| IBIS file stm32u375_385_lqfp100.ibs
[IBIS ver] 4.2
[File name] stm32u375_385_lqfp100.ibs
[File Rev] 1.2
[Date] 23-06-2025
[Source] Data Created at STMicroelectronics
[Notes]  File originated from ELDO simulations.
[Disclaimer]  This information is for modeling purpose only and is
   not guaranted. The information is subject to change without
   notice.
[Copyright] Copyright 2025 STMicroelectronics Inc.
|   Component stm32u375_385_lqfp100
[Component] stm32u375_385_lqfp100
[Manufacturer] STMicroelectronics
[Package]
| variable   typ   min   max
R_pkg  0  NA  NA
L_pkg  0  NA  NA
C_pkg  0  NA  NA
[Pin]   signal_name   model_name
1  PE2  io8_ft_100m
2  PE3  io8_ft_100m_hslv
3  PE4  io8_ft_100m
4  PE5  io8_ft_100m
5  PE6  io8_ft_100m
6  VBAT  power
7  PC13  io8_ft_100m_v33
8  PC14-OSC32_IN  io_ft_tamp
9  PC15-OSC32_OUT  io_ft_tamp
10  VSS  gnd
11  VDD  power
12  PH0-OSC_IN  io8_ft_100m
13  PH1-OSC_OUT  io8_ft_100m
14  NRST  ioreset_v33
15  PC0  io8_ft_100m_hslv
16  PC1  io8_ft_100m_hslv
17  PC2  io8_ft_100m_hslv
18  PC3  io8_ft_100m_hslv
19  VSSA  nc
20  VREFM  nc
21  VREFP  nc
22  VDDA  nc
23  PA0  io8_ft_100m
24  PA1  io8_ft_100m_hslv
25  PA2  io8_ft_100m_hslv
26  PA3  io8_ft_100m_hslv
27  VSS  gnd
28  VDD  power
29  PA4  io8_ft_100m_hslv
30  PA5  io8_ft_100m
31  PA6  io8_ft_100m_hslv
32  PA7  io8_ft_100m_hslv
33  PC4  io8_ft_100m_hslv
34  PC5  io8_ft_100m
35  PB0  io8_ft_100m_hslv
36  PB1  io8_ft_100m_hslv
37  PB2  io8_ft_100m_hslv
38  PE7  io8_ft_100m
39  PE8  io8_ft_100m
40  PE9  io8_ft_100m_hslv
41  PE10  io8_ft_100m_hslv
42  PE11  io8_ft_100m_hslv
43  PE12  io8_ft_100m_hslv
44  PE13  io8_ft_100m_hslv
45  PE14  io8_ft_100m_hslv
46  PE15  io8_ft_100m_hslv
47  PB10  io8_ft_100m_hslv
48  VCAP  nc
49  VSS  gnd
50  VDD  power
51  PB12  io8_ft_100m_hslv
52  PB13  io8_ft_100m_hslv
53  PB14  io8_ft_100m_hslv
54  PB15  io8_ft_100m
55  PD8  io8_ft_100m
56  PD9  io8_ft_100m
57  PD10  io8_ft_100m
58  PD11  io8_ft_100m
59  PD12  io8_ft_100m_hslv
60  PD13  io8_ft_100m_hslv
61  PD14  io8_ft_100m
62  PD15  io8_ft_100m
63  PC6  io8_ft_100m_hslv
64  PC7  io8_ft_100m_hslv
65  PC8  io8_ft_100m_hslv
66  PC9  io8_ft_100m_hslv
67  PA8  io8_ft_100m_hslv
68  PA9  io8_ft_100m
69  PA10  io8_ft_100m
70  PA11  io8usb_ft_phy
71  PA12  io8usb_ft_phy
72  PA13  io8_ft_100m
73  VDDUSB  power
74  VSS  gnd
75  VDD  power
76  PA14  io8_ft_100m
77  PA15  io8_ft_100m
78  PC10  io8_ft_100m_hslv
79  PC11  io8_ft_100m_hslv
80  PC12  io8_ft_100m_hslv
81  PD0  io8_ft_100m
82  PD1  io8_ft_100m
83  PD2  io8_ft_100m_hslv
84  PD3  io8_ft_100m_hslv
85  PD4  io8_ft_100m_hslv
86  PD5  io8_ft_100m_hslv
87  PD6  io8_ft_100m_hslv
88  PD7  io8_ft_100m_hslv
89  PB3  io8_ft_100m_hslv
90  PB4  io8_ft_100m_hslv
91  PB5  io8_ft_100m_hslv
92  PB6  io8_ft_100m_hslv
93  PB7  io8_ft_100m_hslv
94  PH3-BOOT0  io8_ft_100m_hslv
95  PB8  io8_ft_100m_hslv
96  PB9  io8_ft_100m_hslv
97  PE0  io8_ft_100m
98  PE1  io8_ft_100m
99  VSS  gnd
100  VDD  power
[Package Model]   454-lqfp-14x14-100-ldo-250417
[Pin Mapping]   pulldown_ref   pullup_ref   | Comment
1  gndio  vddio
2  gndio  vddio
3  gndio  vddio
4  gndio  vddio
5  gndio  vddio
6  nc  vsw
7  gndio  vsw
8  gndio  vsw
9  gndio  vsw
10  gndio  nc
11  nc  vddio
12  gndio  vddio
13  gndio  vddio
14  gndio  vddio
15  gndio  vddio
16  gndio  vddio
17  gndio  vddio
18  gndio  vddio
19  nc  nc
20  nc  nc
21  nc  nc
22  nc  nc
23  gndio  vddio
24  gndio  vddio
25  gndio  vddio
26  gndio  vddio
27  gndio  nc
28  nc  vddio
29  gndio  vddio
30  gndio  vddio
31  gndio  vddio
32  gndio  vddio
33  gndio  vddio
34  gndio  vddio
35  gndio  vddio
36  gndio  vddio
37  gndio  vddio
38  gndio  vddio
39  gndio  vddio
40  gndio  vddio
41  gndio  vddio
42  gndio  vddio
43  gndio  vddio
44  gndio  vddio
45  gndio  vddio
46  gndio  vddio
47  gndio  vddio
48  nc  nc
49  gndio  nc
50  nc  vddio
51  gndio  vddio
52  gndio  vddio
53  gndio  vddio
54  gndio  vddio
55  gndio  vddio
56  gndio  vddio
57  gndio  vddio
58  gndio  vddio
59  gndio  vddio
60  gndio  vddio
61  gndio  vddio
62  gndio  vddio
63  gndio  vddio
64  gndio  vddio
65  gndio  vddio
66  gndio  vddio
67  gndio  vddio
68  gndio  vddio
69  gndio  vddio
70  gndio  vddusb  | Depending on IO usage
| 70  gndio  vddio  | Depending on IO usage
71  gndio  vddusb  | Depending on IO usage
| 71  gndio  vddio  | Depending on IO usage
72  gndio  vddio
73  nc  vddusb
74  gndio  nc
75  nc  vddio
76  gndio  vddio
77  gndio  vddio
78  gndio  vddio
79  gndio  vddio
80  gndio  vddio
81  gndio  vddio
82  gndio  vddio
83  gndio  vddio
84  gndio  vddio
85  gndio  vddio
86  gndio  vddio
87  gndio  vddio
88  gndio  vddio
89  gndio  vddio
90  gndio  vddio
91  gndio  vddio
92  gndio  vddio
93  gndio  vddio
94  gndio  vddio
95  gndio  vddio
96  gndio  vddio
97  gndio  vddio
98  gndio  vddio
99  gndio  nc
100  nc  vddio
|[Diff Pin]  inv_pin  vdiff  tdelay_typ  tdelay_min  tdelay_max
|71  70  NA  NA  NA  NA
[Model Selector] io8_ft_100m
io8_ft_100m_ls_1v2  "GPIO 100MHz - 5V tolerant - low speed - 1.2V range"
io8_ft_100m_ls_1v8  "GPIO 100MHz - 5V tolerant - low speed - 1.8V range"
io8_ft_100m_ls_3v3  "GPIO 100MHz - 5V tolerant - low speed - 3.3V range"
io8_ft_100m_ms_1v2  "GPIO 100MHz - 5V tolerant - med speed - 1.2V range"
io8_ft_100m_ms_1v8  "GPIO 100MHz - 5V tolerant - med speed - 1.8V range"
io8_ft_100m_ms_3v3  "GPIO 100MHz - 5V tolerant - med speed - 3.3V range"
io8_ft_100m_fs_1v2  "GPIO 100MHz - 5V tolerant - fast speed - 1.2V range"
io8_ft_100m_fs_1v8  "GPIO 100MHz - 5V tolerant - fast speed - 1.8V range"
io8_ft_100m_fs_3v3  "GPIO 100MHz - 5V tolerant - fast speed - 3.3V range"
io8_ft_100m_hs_1v2  "GPIO 100MHz - 5V tolerant - high speed - 1.2V range"
io8_ft_100m_hs_1v8  "GPIO 100MHz - 5V tolerant - high speed - 1.8V range"
io8_ft_100m_hs_3v3  "GPIO 100MHz - 5V tolerant - high speed - 3.3V range"
[Model Selector] io8_ft_100m_hslv
io8_ft_100m_ls_1v2  "GPIO 100MHz - 5V tolerant - low speed - 1.2V range"
io8_ft_100m_ls_1v8  "GPIO 100MHz - 5V tolerant - low speed - 1.8V range"
io8_ft_100m_ls_3v3  "GPIO 100MHz - 5V tolerant - low speed - 3.3V range"
io8_ft_100m_ms_1v2  "GPIO 100MHz - 5V tolerant - med speed - 1.2V range"
io8_ft_100m_ms_1v8  "GPIO 100MHz - 5V tolerant - med speed - 1.8V range"
io8_ft_100m_ms_3v3  "GPIO 100MHz - 5V tolerant - med speed - 3.3V range"
io8_ft_100m_fs_1v2  "GPIO 100MHz - 5V tolerant - fast speed - 1.2V range"
io8_ft_100m_fs_1v8  "GPIO 100MHz - 5V tolerant - fast speed - 1.8V range"
io8_ft_100m_fs_3v3  "GPIO 100MHz - 5V tolerant - fast speed - 3.3V range"
io8_ft_100m_hs_1v2  "GPIO 100MHz - 5V tolerant - high speed - 1.2V range"
io8_ft_100m_hs_1v8  "GPIO 100MHz - 5V tolerant - high speed - 1.8V range"
io8_ft_100m_hs_3v3  "GPIO 100MHz - 5V tolerant - high speed - 3.3V range"
io8_ft_100m_hslv_ls_1v2  "GPIO 100MHz low voltage optimization - 5V tolerant - low speed - 1.2V range"
io8_ft_100m_hslv_ls_1v8  "GPIO 100MHz low voltage optimization - 5V tolerant - low speed - 1.8V range"
io8_ft_100m_hslv_ls_2v5  "GPIO 100MHz low voltage optimization - 5V tolerant - low speed - 3.3V range"
io8_ft_100m_hslv_ms_1v2  "GPIO 100MHz low voltage optimization - 5V tolerant - med speed - 1.2V range"
io8_ft_100m_hslv_ms_1v8  "GPIO 100MHz low voltage optimization - 5V tolerant - med speed - 1.8V range"
io8_ft_100m_hslv_ms_2v5  "GPIO 100MHz low voltage optimization - 5V tolerant - med speed - 3.3V range"
io8_ft_100m_hslv_fs_1v2  "GPIO 100MHz low voltage optimization - 5V tolerant - fast speed - 1.2V range"
io8_ft_100m_hslv_fs_1v8  "GPIO 100MHz low voltage optimization - 5V tolerant - fast speed - 1.8V range"
io8_ft_100m_hslv_fs_2v5  "GPIO 100MHz low voltage optimization - 5V tolerant - fast speed - 3.3V range"
io8_ft_100m_hslv_hs_1v2  "GPIO 100MHz low voltage optimization - 5V tolerant - high speed - 1.2V range"
io8_ft_100m_hslv_hs_1v8  "GPIO 100MHz low voltage optimization - 5V tolerant - high speed - 1.8V range"
io8_ft_100m_hslv_hs_2v5  "GPIO 100MHz low voltage optimization - 5V tolerant - high speed - 3.3V range"
[Model Selector] io8_ft_100m_v33
io8_ft_100m_v33_ls_1v2  "GPIO_V33 100MHz - 5V tolerant - low speed - 1.2V range"
io8_ft_100m_v33_ls_1v8  "GPIO_V33 100MHz - 5V tolerant - low speed - 1.8V range"
io8_ft_100m_v33_ls_3v3  "GPIO_V33 100MHz - 5V tolerant - low speed - 3.3V range"
io8_ft_100m_v33_ms_1v2  "GPIO_V33 100MHz - 5V tolerant - med speed - 1.2V range"
io8_ft_100m_v33_ms_1v8  "GPIO_V33 100MHz - 5V tolerant - med speed - 1.8V range"
io8_ft_100m_v33_ms_3v3  "GPIO_V33 100MHz - 5V tolerant - med speed - 3.3V range"
io8_ft_100m_v33_fs_1v2  "GPIO_V33 100MHz - 5V tolerant - fast speed - 1.2V range"
io8_ft_100m_v33_fs_1v8  "GPIO_V33 100MHz - 5V tolerant - fast speed - 1.8V range"
io8_ft_100m_v33_fs_3v3  "GPIO_V33 100MHz - 5V tolerant - fast speed - 3.3V range"
io8_ft_100m_v33_hs_1v2  "GPIO_V33 100MHz - 5V tolerant - high speed - 1.2V range"
io8_ft_100m_v33_hs_1v8  "GPIO_V33 100MHz - 5V tolerant - high speed - 1.8V range"
io8_ft_100m_v33_hs_3v3  "GPIO_V33 100MHz - 5V tolerant - high speed - 3.3V range"
[Model Selector] io8usb_ft_phy
io8_ft_100m_ls_1v2  "GPIO 100MHz - 5V tolerant - low speed - 1.2V range"
io8_ft_100m_ls_1v8  "GPIO 100MHz - 5V tolerant - low speed - 1.8V range"
io8_ft_100m_ls_3v3  "GPIO 100MHz - 5V tolerant - low speed - 3.3V range"
io8_ft_100m_ms_1v2  "GPIO 100MHz - 5V tolerant - med speed - 1.2V range"
io8_ft_100m_ms_1v8  "GPIO 100MHz - 5V tolerant - med speed - 1.8V range"
io8_ft_100m_ms_3v3  "GPIO 100MHz - 5V tolerant - med speed - 3.3V range"
io8_ft_100m_fs_1v2  "GPIO 100MHz - 5V tolerant - fast speed - 1.2V range"
io8_ft_100m_fs_1v8  "GPIO 100MHz - 5V tolerant - fast speed - 1.8V range"
io8_ft_100m_fs_3v3  "GPIO 100MHz - 5V tolerant - fast speed - 3.3V range"
io8_ft_100m_hs_1v2  "GPIO 100MHz - 5V tolerant - high speed - 1.2V range"
io8_ft_100m_hs_1v8  "GPIO 100MHz - 5V tolerant - high speed - 1.8V range"
io8_ft_100m_hs_3v3  "GPIO 100MHz - 5V tolerant - high speed - 3.3V range"
io8usb_ft_phy_hs_3v3   "USB full speed"
io8usb_ft_phy_ls_3v3   "USB low speed"
[Model Selector] io_ft_tamp
io_ft_tamp_ls_1v2 "io8_ft tamp low speed @ 1.2V"
io_ft_tamp_ls_1v8 "io8_ft tamp low speed @ 1.8V"
io_ft_tamp_ls_3v3 "io8_ft tamp low speed @ 3.3V"
io_ft_tamp_ms_1v2 "io8_ft tamp med speed @ 1.2V"
io_ft_tamp_ms_1v8 "io8_ft tamp med speed @ 1.8V"
io_ft_tamp_ms_3v3 "io8_ft tamp med speed @ 3.3V"
io_ft_tamp_fs_1v2 "io8_ft tamp fast speed @ 1.2V"
io_ft_tamp_fs_1v8 "io8_ft tamp fast speed @ 1.8V"
io_ft_tamp_fs_3v3 "io8_ft tamp fast speed @ 3.3V"
io_ft_tamp_hs_1v2 "io8_ft tamp high speed @ 1.2V"
io_ft_tamp_hs_1v8 "io8_ft tamp high speed @ 1.8V"
io_ft_tamp_hs_3v3 "io8_ft tamp high speed @ 3.3V"
[Model Selector] ioreset_v33
ioreset_v33_1v2 "Reset PAD. 5V tolerant. 1.2V range"
ioreset_v33_1v8 "Reset PAD. 5V tolerant. 1.8V range"
ioreset_v33_3v3 "Reset PAD. 5V tolerant. 3.3V range"
[Define Package Model]  454-lqfp-14x14-100-ldo-250417
[Manufacturer]  Unknown
[OEM]  Unknown
[Description]  None
[Number Of Pins]  96
[Pin Numbers]
| Pin Num   Terminal Name
14 | NRST
23 | PA0
69 | PA10
70 | PA11
71 | PA12
72 | PA13
76 | PA14
77 | PA15
24 | PA1
25 | PA2
26 | PA3
29 | PA4
30 | PA5
31 | PA6
32 | PA7
67 | PA8
68 | PA9
35 | PB0
47 | PB10
51 | PB12
52 | PB13
53 | PB14
54 | PB15
36 | PB1
37 | PB2
89 | PB3
90 | PB4
91 | PB5
92 | PB6
93 | PB7
95 | PB8
96 | PB9
15 | PC0
78 | PC10
79 | PC11
80 | PC12
7 | PC13
8 | PC14-OSC32_IN
9 | PC15-OSC32_OUT
16 | PC1
17 | PC2
18 | PC3
33 | PC4
34 | PC5
63 | PC6
64 | PC7
65 | PC8
66 | PC9
81 | PD0
57 | PD10
58 | PD11
59 | PD12
60 | PD13
61 | PD14
62 | PD15
82 | PD1
83 | PD2
84 | PD3
85 | PD4
86 | PD5
87 | PD6
88 | PD7
55 | PD8
56 | PD9
97 | PE0
41 | PE10
42 | PE11
43 | PE12
44 | PE13
45 | PE14
46 | PE15
98 | PE1
1 | PE2
2 | PE3
3 | PE4
4 | PE5
5 | PE6
38 | PE7
39 | PE8
40 | PE9
12 | PH0-OSC_IN
13 | PH1-OSC_OUT
94 | PH3-BOOT0
48 | VCAP
6 | VBAT
50 | VDD
75 | VDD
100 | VDD
28 | VDD
11 | VDD
22 | VDDA
73 | VDDUSB
20 | VREFM
21 | VREFP
10 | VSS
19 | VSSA
|[Merged Pins]  10
|27  |  VSS
|49  |  VSS
|74  |  VSS
|99  |  VSS
[Model Data]
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[End Model Data]
[End Package Model]
|End [Component]
| Models and submodels in the file (53): io8_ft_100m_fs_1v2 (I/O), io8_ft_100m_fs_1v8 (I/O), io8_ft_100m_fs_3v3 (I/O), io8_ft_100m_hs_1v2 (I/O), io8_ft_100m_hs_1v8 (I/O), io8_ft_100m_hs_3v3 (I/O), io8_ft_100m_hslv_fs_1v2 (I/O), io8_ft_100m_hslv_fs_1v8 (I/O), io8_ft_100m_hslv_fs_2v5 (I/O), io8_ft_100m_hslv_hs_1v2 (I/O), io8_ft_100m_hslv_hs_1v8 (I/O), io8_ft_100m_hslv_hs_2v5 (I/O), io8_ft_100m_hslv_ls_1v2 (I/O), io8_ft_100m_hslv_ls_1v8 (I/O), io8_ft_100m_hslv_ls_2v5 (I/O), io8_ft_100m_hslv_ms_1v2 (I/O), io8_ft_100m_hslv_ms_1v8 (I/O), io8_ft_100m_hslv_ms_2v5 (I/O), io8_ft_100m_ls_1v2 (I/O), io8_ft_100m_ls_1v8 (I/O), io8_ft_100m_ls_3v3 (I/O), io8_ft_100m_ms_1v2 (I/O), io8_ft_100m_ms_1v8 (I/O), io8_ft_100m_ms_3v3 (I/O), io8_ft_100m_v33_fs_1v2 (I/O), io8_ft_100m_v33_fs_1v8 (I/O), io8_ft_100m_v33_fs_3v3 (I/O), io8_ft_100m_v33_hs_1v2 (I/O), io8_ft_100m_v33_hs_1v8 (I/O), io8_ft_100m_v33_hs_3v3 (I/O), io8_ft_100m_v33_ls_1v2 (I/O), io8_ft_100m_v33_ls_1v8 (I/O), io8_ft_100m_v33_ls_3v3 (I/O), io8_ft_100m_v33_ms_1v2 (I/O), io8_ft_100m_v33_ms_1v8 (I/O), io8_ft_100m_v33_ms_3v3 (I/O), io8usb_ft_phy_hs_3v3 (I/O), io8usb_ft_phy_ls_3v3 (I/O), io_ft_tamp_fs_1v2 (I/O), io_ft_tamp_fs_1v8 (I/O), io_ft_tamp_fs_3v3 (I/O), io_ft_tamp_hs_1v2 (I/O), io_ft_tamp_hs_1v8 (I/O), io_ft_tamp_hs_3v3 (I/O), io_ft_tamp_ls_1v2 (I/O), io_ft_tamp_ls_1v8 (I/O), io_ft_tamp_ls_3v3 (I/O), io_ft_tamp_ms_1v2 (I/O), io_ft_tamp_ms_1v8 (I/O), io_ft_tamp_ms_3v3 (I/O), ioreset_v33_1v2 (I/O_open_drain), ioreset_v33_1v8 (I/O_open_drain), ioreset_v33_3v3 (I/O_open_drain)
